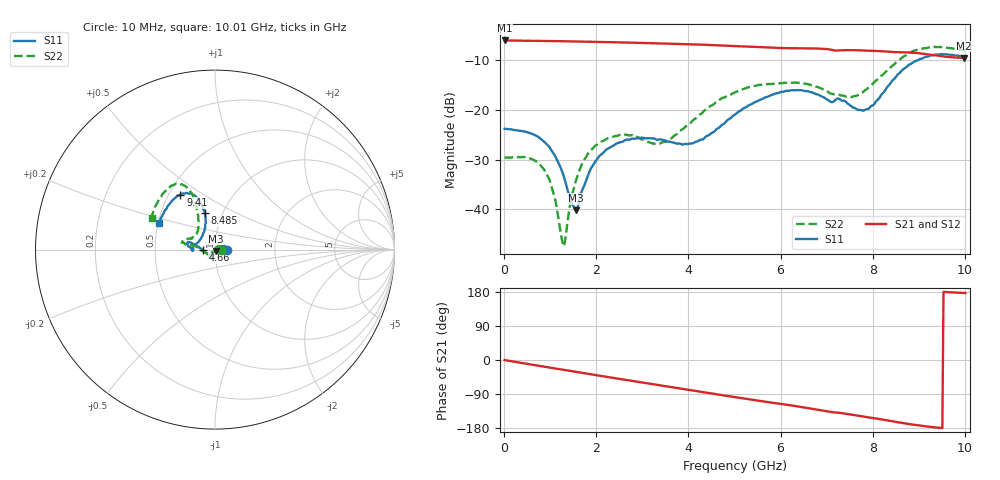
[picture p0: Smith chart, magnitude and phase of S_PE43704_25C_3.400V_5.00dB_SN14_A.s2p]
! Device ID: PE43704
! Dir: z:\PE43704\PE43704_Char_1_20130516\PE43704\AMB\3p400V\5p00dB
! Serial: 14
! Insertion: A
! Impedance: 50 ohm
! Temp: Amb
! VDD: 3.400V
! Attenuation Step: 5.00dB
! IDD: 1.141121e-01mA
#  Hz  S  RI  R  50
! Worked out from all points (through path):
!   401 points, 10 MHz to 10.01 GHz, reference 50 ohm
!   highest |S21| = -5.99 dB at 10 MHz (marker M1); lowest = -9.5 dB at 9.985 GHz (marker M2)
!   group delay of S21, straight-line fit = 52.3 ps
!   lowest |S11| = -40.2 dB at 1.56 GHz (marker M3), VSWR 1.02, Z = 50.6 - j0.762 ohm
!   |S11| at or under -10 dB: start of sweep to 8.968 GHz
!   |S22| runs from -47.4 to -7.3 dB; largest |S21 - S12| = 0.0035
!   S11 on the Smith chart (normalised r, x): 10 MHz: 1.14, +0.00; 4.66 GHz: 0.88, -0.01; 8.485 GHz: 0.83, +0.35; 9.41 GHz: 0.57, +0.40; 10.01 GHz: 0.51, +0.17
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1e7  0.0647 0.000202  0.5015 -0.00208  0.5018 -0.00202  0.0331 0.000347
5.6e8  0.0552 0.0199  0.4875 -0.0985  0.4875 -0.0984  0.0261 0.0197
8.6e8  0.0436 0.0208  0.4727 -0.1482  0.4728 -0.1481  0.0168 0.0191
1.06e9  0.0336 0.0158  0.4605 -0.1803  0.4606 -0.18  0.00768 0.0129
1.285e9  0.0213 0.00639  0.443 -0.2152  0.4431 -0.215  -0.0033 0.00272
1.56e9  0.00628 -0.00753  0.4188 -0.255  0.4188 -0.2549  -0.0143 -0.0134
1.685e9  0.00045 -0.0153  0.4064 -0.2725  0.4064 -0.2723  -0.019 -0.0211
1.91e9  -0.0081 -0.0257  0.3819 -0.3015  0.3821 -0.3014  -0.0241 -0.0326
2.235e9  -0.0157 -0.0373  0.3434 -0.3395  0.3437 -0.3393  -0.0295 -0.0425
3.36e9  -0.0215 -0.0458  0.1872 -0.4293  0.1876 -0.4291  -0.0352 -0.0295
4.06e9  -0.037 -0.0277  0.0798 -0.4511  0.0803 -0.451  -0.0756 -0.00381
4.66e9  -0.0663 -0.00391  -0.0121 -0.4471  -0.0117 -0.4471  -0.1228 0.0233
5.01e9  -0.0893 0.0127  -0.0609 -0.4359  -0.0605 -0.4361  -0.1486 0.0254
5.96e9  -0.1434 0.0422  -0.1788 -0.3821  -0.1775 -0.3824  -0.1817 0.0394
6.685e9  -0.1493 0.0193  -0.2606 -0.3251  -0.2608 -0.3248  -0.1693 0.0527
7.46e9  -0.1128 0.0253  -0.3187 -0.2428  -0.3185 -0.2433  -0.1073 0.0845
7.785e9  -0.0807 0.0565  -0.3409 -0.2046  -0.3411 -0.2059  -0.0927 0.1193
8.36e9  -0.0523 0.1722  -0.3633 -0.1302  -0.3625 -0.132  -0.1026 0.2402
8.485e9  -0.0564 0.2032  -0.3671 -0.1121  -0.3653 -0.114  -0.1123 0.2729
9.41e9  -0.1926 0.3049  -0.3525 -0.00843  -0.3525 -0.00717  -0.2545 0.3462
9.985e9  -0.3062 0.1575  -0.3338 0.0181  -0.3349 0.0186  -0.3496 0.186
1.001e10  -0.3113 0.1474  -0.3343 0.018  -0.3368 0.0182  -0.353 0.1775
